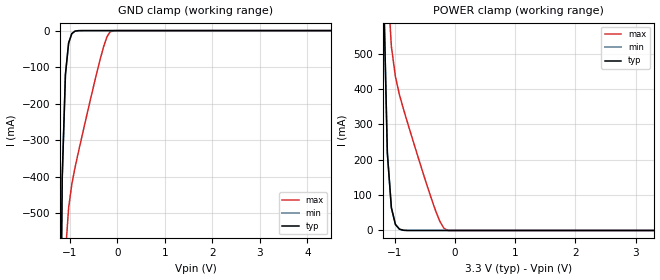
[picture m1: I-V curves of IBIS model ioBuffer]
| IBIS file created by T2B Version 15.0.2.03101 S001
| Cadence Design Systems, Inc. 2011
| Simulator:  ****** HSPICE -- K-2015.06-1 linux64 (Jun 10 2015) ******
[IBIS ver] 3.2
[File name]  f1912-in.ibs
[File Rev]  0.1
[Date]   August 07, 2015
[Source] Integrated Device Technology, Inc.
|   Component f1912
[Component] f1912
[Manufacturer] Integrated Device Technology, Inc.
[Package]
| variable   typ   min   max
R_pkg   2.000m   1.000m   4.000m
L_pkg   0.200nH   0.100nH   0.400nH
C_pkg   2.000pF   1.000pF   4.000pF
[Pin]  signal_name   model_name   R_pin   L_pin   C_pin
in  in   ioBuffer
gnd   gnd   GND
vdd   vdd   POWER
| Models and submodels in the file (1): ioBuffer (Input)
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|   Model ioBuffer
[Model] ioBuffer
Model_type Input
Polarity   Non-Inverting
Vinl =  0.630V
Vinh =  1.170V
C_comp   0.697pF   0.682pF   0.705pF
[Temperature Range]   25.000   0.105k   -40.000
[Voltage Range]   3.300V   3.000V   5.250V
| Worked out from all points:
|   GND clamp passes 1 mA (typ) near -0.86 V on its own axis
|   POWER clamp passes 1 mA (typ) near -0.86 V on its own axis
[GND_clamp]
|Voltage   I(typ)   I(min)   I(max)
-3.3V     -159.2A    -158.9A    -160.4A
-1.223V   -1.273A    -1.272A    -1.842A
-1.156V   -400.7mA   -400.6mA   -930.7mA
-1.089V   -120.4mA   -120.3mA   -611.2mA
-1.022V   -34.04mA   -34.02mA   -485.9mA
-955mV    -8.347mA   -8.344mA   -421.4mA
-888mV    -1.536mA   -1.536mA   -375.8mA
-553mV    -5.511uA   -5.889uA   -183.1mA
-352mV    -3.501uA   -3.743uA   -75.39mA
-218mV    -2.168uA   -2.318uA   -17.5mA
-151mV    -1.502uA   -1.605uA   -3.571mA
6.6V      65.97uA    70.5uA     60.82uA
[POWER_clamp]
|Voltage   I(typ)   I(min)   I(max)
-3.3V     159.2A     158.9A     160.4A
-1.189V   713.6mA    713.3mA    1.245A
-1.122V   218.8mA    218.7mA    712.3mA
-1.055V   64.06mA    64.04mA    519.6mA
-988mV    17.09mA    17.08mA    434.7mA
-921mV    3.665mA    3.664mA    383.5mA
-586mV    34.97nA    35.23nA    193.1mA
-318mV    1.348nA    1.4nA      54.5mA
-251mV    668pA      695pA      26.03mA
-184mV    221pA      230pA      6.489mA
-117mV    0A         0A         0A
3.3V      0A         0A         0A
